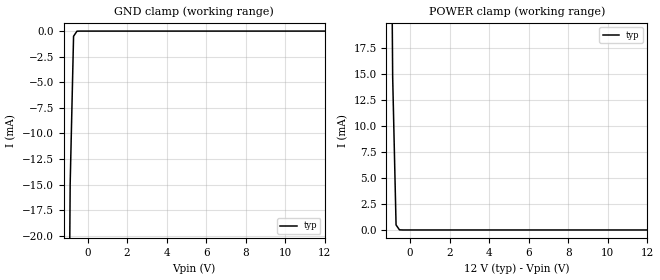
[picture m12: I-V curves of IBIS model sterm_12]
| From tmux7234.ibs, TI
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| sterm_12
[Model]   sterm_12
Model_type   Terminator
|   typ   min   max
C_comp   6.362683e-12   NA   NA
[Voltage Range]   12   NA   NA
[Temperature Range]   27   NA   NA
[Power Clamp Reference]   12   NA   NA
[GND Clamp Reference]   0   NA   NA
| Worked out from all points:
|   GND clamp passes 1 mA (typ) near -0.71 V on its own axis
|   POWER clamp passes 1 mA (typ) near -0.71 V on its own axis
[GND Clamp]
|   Voltage   I(typ)   I(min)   I(max)
-5V       -2.118A    NA         NA
-1.051V   -61.67mA   NA         NA
-878.8mV  -14.96mA   NA         NA
-707.1mV  -503.4uA   NA         NA
-535.4mV  -9.8uA     NA         NA
12V       344.9pA    NA         NA
[POWER Clamp]
|   Voltage   I(typ)   I(min)   I(max)
-5V       2.743A     NA         NA
-1.05V    57.03mA    NA         NA
-878.8mV  14.74mA    NA         NA
-707.1mV  485.1uA    NA         NA
-535.4mV  12.3uA     NA         NA
12V       -348.9pA   NA         NA
